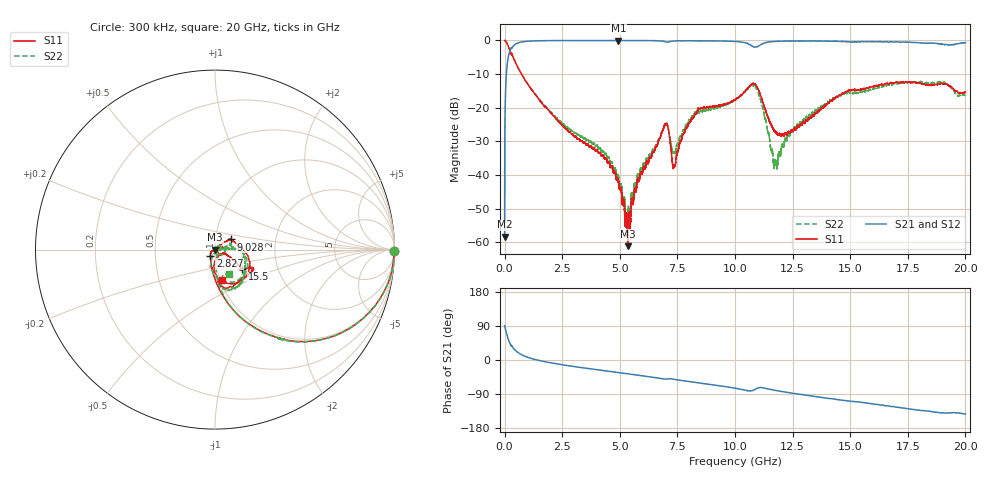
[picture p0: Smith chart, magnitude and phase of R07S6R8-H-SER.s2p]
!{R07S6R8}
!Johanson Technology Inc.
!www.johansontechnology.com
!Test Board Conditions:
!Substrate Type  RO4350B
!Substrate Thickness  10 mil
!Substrate Dk  3.66
!TL Type: GCPW
!TL Trace Width  21 mil
!TL Gap  20 mil
!Electrode orientation  Horizontal
!DUT TOPOLOGY	SERIES
!Mounting Pad LxW  16x21 mil
! Created Sat Feb  6 11:38:31 2021
# hz S ma R 50
! 2 Port Network Data from SP1.SP block
! freq  magS11  angS11  magS21  angS21  magS12  angS12  magS22  angS22
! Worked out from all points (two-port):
!   20001 points, 300 kHz to 20 GHz, reference 50 ohm
!   highest |S21| = -0.02 dB at 4.937 GHz (marker M1); lowest = -58.3 dB at 300 kHz (marker M2)
!   |S21| within 3 dB of the highest: 233.1 MHz to end of sweep
!   lowest |S11| = -61.1 dB at 5.349 GHz (marker M3), VSWR 1.00, Z = 50 - j0.0825 ohm
!   |S11| at or under -10 dB: 731 MHz to end of sweep
!   |S22| runs from -56.1 to 0.0 dB; largest |S21 - S12| = 0.013
!   S11 on the Smith chart (normalised r, x): 300 kHz: open; 2.827 GHz: 0.95, -0.07; 9.028 GHz: 1.19, +0.14; 15.5 GHz: 1.32, -0.30; 20 GHz: 1.02, -0.35
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300000  0.999 -0.5  0.001218 90.8  0.001324 87.2  0.9987 -0.4
1.093e8  0.9028 -25.9  0.4255 64.3  0.4258 64.3  0.9029 -25.9
2.813e8  0.6303 -52.7  0.7681 37.9  0.7678 37.8  0.6333 -52.8
9.043e8  0.2523 -81.0  0.9659 9.3  0.966 9.3  0.2542 -79.9
2.8273e9  0.04387 -126.2  0.996 -15.7  0.995 -15.6  0.04857 -79.1
3.3343e9  0.03212 -138.7  0.9957 -20.1  0.9963 -20.1  0.03712 -73.7
4.9373e9  0.007845 -146.8  0.998 -33.3  0.9966 -33.3  0.009632 -67.8
5.3493e9  0.0008778 -69.9  0.9956 -36.6  0.9954 -36.7  0.002769 3.3
5.8333e9  0.008314 10.0  0.995 -40.5  0.9951 -40.5  0.00916 71.6
6.6673e9  0.03138 28.5  0.989 -47.7  0.989 -47.8  0.03268 38.0
7.0293e9  0.05697 -15.3  0.9451 -50.3  0.9467 -50.3  0.05859 -16.8
7.3633e9  0.01378 2.3  0.9821 -51.0  0.9825 -51.0  0.02105 -10.7
8.0683e9  0.06188 40.2  0.9889 -57.4  0.9897 -57.4  0.06627 15.7
9.0283e9  0.1051 32.5  0.9834 -65.3  0.9837 -65.5  0.09806 10.1
1.00003e10  0.1318 11.4  0.9673 -74.4  0.9675 -74.4  0.1296 -0.8
1.09113e10  0.2177 -60.8  0.7966 -76.2  0.7958 -76.0  0.1973 -66.8
1.17593e10  0.04376 -70.0  0.9696 -80.3  0.9689 -80.3  0.01589 -48.5
1.23683e10  0.04226 -33.4  0.9784 -86.5  0.9794 -86.5  0.03911 6.1
1.33343e10  0.07361 -22.8  0.981 -95.0  0.9816 -95.0  0.08163 2.4
1.54983e10  0.1867 -35.9  0.9618 -111.8  0.9577 -111.7  0.1717 -17.0
1.66673e10  0.2261 -26.0  0.946 -121.1  0.9508 -121.6  0.2176 -42.4
2e10  0.1719 -76.1  0.93 -142.7  0.9254 -142.7  0.16 -60.4
